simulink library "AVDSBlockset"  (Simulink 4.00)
undefined symbols (not defined in the file or in its folder): SimulinkConfiguration, SimulinkData, SimulinkVehicle01
libraries: simulink3 x7

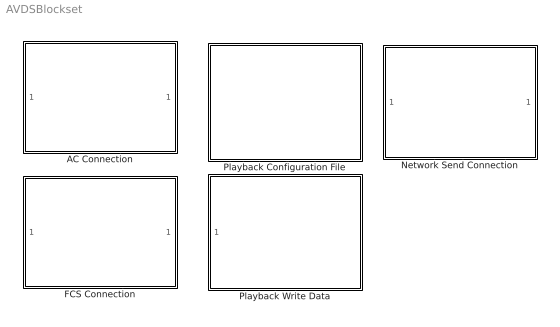
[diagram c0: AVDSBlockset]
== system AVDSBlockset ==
  AC Connection : Subsystem  Description=This block is used to connect Simulink to AVDS through the MATLAB AC model.  mask(AC Connection Block){RealTime=on}
      mask prompts: RealTime "Real Time Operation"
      mask help: This block connects a Simulink vehicle simulation to AVDS through shared memory. See help for more information.
  FCS Connection : Subsystem  Description=This block is used to connect Simulink to AVDS through the MATLAB AC model.
  Network Send Connection : Subsystem  Description=This block is used to connect Simulink to AVDS through the MATLAB AC model.  mask(Network Send Connection Block){VehicleHandleName=SimulinkVehicle01, TransmitRateHz=20, CraftType=1, InitLatitudeDeg=37.981523, InitLongitudeDeg=-122.063400, InitAltitudeFeet=10000, RealTime=on}
      mask prompts: VehicleHandleName "Vehicle Handle Name (up to 28 characters)"; TransmitRateHz "Transmit Rate (Hz)"; CraftType "Craft Type Index"; InitLatitudeDeg "Initial Latitude (Degrees Decimal)"; InitLongitudeDeg "Initial Longitude (Degrees Decimal) ( west longitude = negative)"; InitAltitudeFeet "Initial Altitude (Feet)"; RealTime "Real Time"
      mask help: Sends AVDS vehicle packets to the local network from Matlab using multicast network functions. See help for more information.
  Playback Configuration File : Subsystem  mask(Playback Configuration File Block){ConfigurationFileName=SimulinkConfiguration.ply.ini, DataFileNameBase=SimulinkData, NumberVehicles=10}
      mask prompts: ConfigurationFileName "Playback Configuration File Name"; DataFileNameBase "Data File Name Base (files use this name plus 2 digits)"; NumberVehicles "Number of Vehicles"
      mask help: This function writes an initialization file that configures AVDS playback. See help for more information.
  Playback Write Data : Subsystem  mask(Save Playback Data Block){DataFileNameBase=SimulinkData, VehicleID=01, NumberDataSignals=7}
      mask prompts: DataFileNameBase "Data File Name Base (files use this name plus the 2 digit ID)"; VehicleID "Vehicle ID (less than total number of vehicles)"; NumberDataSignals "Number Data Signals (number inputs to block)"
      mask help: Used to manage data for output to an AVDS playback file. See help for more information.

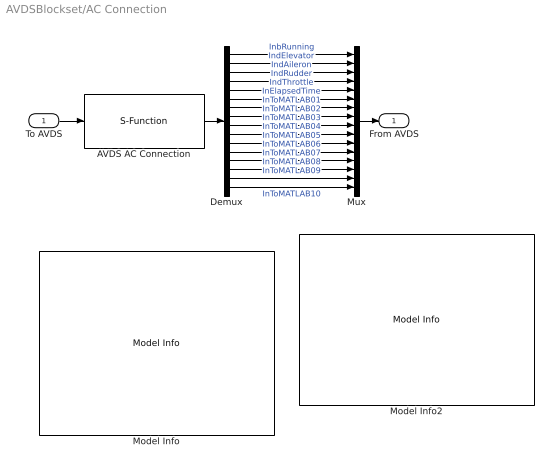
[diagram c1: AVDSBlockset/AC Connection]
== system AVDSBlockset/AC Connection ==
  To AVDS : Inport  Port=1  LatchInput=off
  AVDS AC Connection : S-Function  FunctionName=AVDSSimulationBlock  Parameters=3,25,4,16,RealTime  PortCounts=[]  SFunctionModules=''
  Demux : Demux  Outputs=16  BusSelectionMode=off
  Model Info : simulink3/Signals & Systems/Model Info  InitialBlockCM=none  BlockCM=none  Frame=off  DisplayStringWithTags=|  HorizontalTextAlignment=Left  LeftAlignmentValue=0.02  SourceBlockDiagram=AVDSBlockset  TagMaxNumber=20
      | Block Inputs:
      | OutPositionX, OutPositionY, OutPositionZ
      | OutRotationX, OutRotationY,OutRotationZ
      | OutAlpha, OutBeta
      | OutG
      | OutVelocity
      | OutM
      | OutDeltaRudde, OutDeltaElevator, OutDeltaAileron  
      | OutEngine
      | OutToAVDS01,  OutToAVDS02, OutToAVDS03
      | OutToAVDS04,  OutToAVDS05, OutToAVDS06,
      |  OutToAVDS07, OutToAVDS08,  OutToAVDS09,
      | OutToAVDS10
  Model Info2 : simulink3/Signals & Systems/Model Info  InitialBlockCM=none  BlockCM=none  Frame=off  DisplayStringWithTags=|  HorizontalTextAlignment=Left  LeftAlignmentValue=0.02  SourceBlockDiagram=AVDSBlockset  TagMaxNumber=20
      | BlockOutputs:
      | InbRunning
      | IndElevator, IndAileron, IndRudder, IndThrottle
      | InElapsedTime
      | InToMATLAB01, InToMATLAB02, InToMATLAB03
      | InToMATLAB04, InToMATLAB05, InToMATLAB06
      | InToMATLAB07, InToMATLAB08, InToMATLAB09
      | InToMATLAB10
  Mux : Mux  Inputs=16
  From AVDS : Outport  Port=1
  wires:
  To AVDS/1 -> AVDS AC Connection/1
  AVDS AC Connection/1 -> Demux/1
  Demux/1 -> Mux/1  "InbRunning"
  Demux/2 -> Mux/2  "IndElevator"
  Demux/3 -> Mux/3  "IndAileron"
  Demux/4 -> Mux/4  "IndRudder"
  Demux/5 -> Mux/5  "IndThrottle"
  Demux/6 -> Mux/6  "InElapsedTime"
  Demux/7 -> Mux/7  "InToMATLAB01"
  Demux/8 -> Mux/8  "InToMATLAB02"
  Demux/9 -> Mux/9  "InToMATLAB03"
  Demux/10 -> Mux/10  "InToMATLAB04"
  Demux/11 -> Mux/11  "InToMATLAB05"
  Demux/12 -> Mux/12  "InToMATLAB06"
  Demux/13 -> Mux/13  "InToMATLAB07"
  Demux/14 -> Mux/14  "InToMATLAB08"
  Demux/15 -> Mux/15  "InToMATLAB09"
  Demux/16 -> Mux/16  "InToMATLAB10"
  Mux/1 -> From AVDS/1

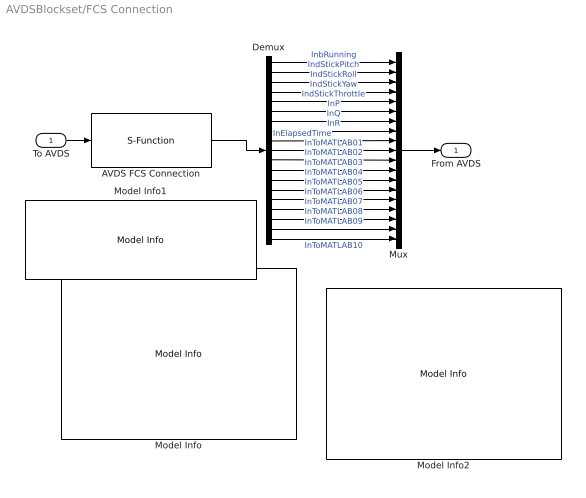
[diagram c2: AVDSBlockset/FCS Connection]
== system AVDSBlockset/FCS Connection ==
  To AVDS : Inport  Port=1  LatchInput=off
  AVDS FCS Connection : S-Function  FunctionName=AVDSSimulationBlock  Parameters=1,14,2,19  PortCounts=[]  SFunctionModules=''
  Demux : Demux  Outputs=19  BusSelectionMode=off
  Model Info : simulink3/Signals & Systems/Model Info  InitialBlockCM=none  BlockCM=none  Frame=off  DisplayStringWithTags=|  HorizontalTextAlignment=Left  LeftAlignmentValue=0.02  SourceBlockDiagram=AVDSBlockset  TagMaxNumber=20
      | Block Inputs:
      | 
      | OutPositionX, OutPositionY, OutPositionZ
      | OutRotationX, OutRotationY,OutRotationZ
      | OutAlpha, OutBeta
      | OutG
      | OutVelocity
      | OutM
      | OutDeltaRudde, OutDeltaElevator, OutDeltaAileron  
      | OutEngine
      | OutToAVDS01,  OutToAVDS02, OutToAVDS03
      | OutToAVDS04,  OutToAVDS05, OutToAVDS06,
      |  OutToAVDS07, OutToAVDS08,  OutToAVDS09,
      | OutToAVDS10
  Model Info1 : simulink3/Signals & Systems/Model Info  InitialBlockCM=none  BlockCM=none  Frame=off  DisplayStringWithTags=|  HorizontalTextAlignment=Left  LeftAlignmentValue=0.02  SourceBlockDiagram=AVDSBlockset  TagMaxNumber=20
      | AVDS AC Connection Block
      | 
      | Version %<ModelVersion>
      | Revision Date: %<LastModificationDate>
  Model Info2 : simulink3/Signals & Systems/Model Info  InitialBlockCM=none  BlockCM=none  Frame=off  DisplayStringWithTags=|  HorizontalTextAlignment=Left  LeftAlignmentValue=0.02  SourceBlockDiagram=AVDSBlockset  TagMaxNumber=20
      | BlockOutputs:
      | 
      | InbRunning
      | IndElevator, IndAileron, IndRudder, IndThrottle
      | InElapsedTime
      | InToMATLAB01, InToMATLAB02, InToMATLAB03
      | InToMATLAB04, InToMATLAB05, InToMATLAB06
      | InToMATLAB07, InToMATLAB08, InToMATLAB09
      | InToMATLAB10
  Mux : Mux  Inputs=19
  From AVDS : Outport  Port=1
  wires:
  AVDS FCS Connection/1 -> Demux/1
  To AVDS/1 -> AVDS FCS Connection/1
  Mux/1 -> From AVDS/1
  Demux/14 -> Mux/14  "InToMATLAB05"
  Demux/13 -> Mux/13  "InToMATLAB04"
  Demux/12 -> Mux/12  "InToMATLAB03"
  Demux/11 -> Mux/11  "InToMATLAB02"
  Demux/10 -> Mux/10  "InToMATLAB01"
  Demux/9 -> Mux/9  "InElapsedTime"
  Demux/8 -> Mux/8  "InR"
  Demux/7 -> Mux/7  "InQ"
  Demux/6 -> Mux/6  "InP"
  Demux/5 -> Mux/5  "IndStickThrottle"
  Demux/4 -> Mux/4  "IndStickYaw"
  Demux/3 -> Mux/3  "IndStickRoll"
  Demux/2 -> Mux/2  "IndStickPitch"
  Demux/1 -> Mux/1  "InbRunning"
  Demux/15 -> Mux/15  "InToMATLAB06"
  Demux/16 -> Mux/16  "InToMATLAB07"
  Demux/17 -> Mux/17  "InToMATLAB08"
  Demux/18 -> Mux/18  "InToMATLAB09"
  Demux/19 -> Mux/19  "InToMATLAB10"

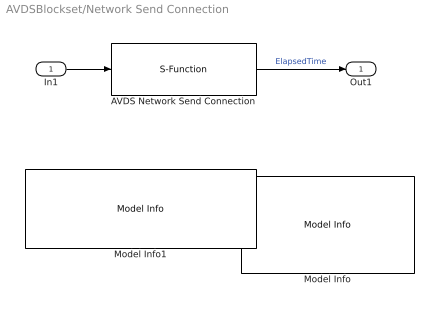
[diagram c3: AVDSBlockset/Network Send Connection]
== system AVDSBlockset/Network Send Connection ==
  In1 : Inport  Port=1  LatchInput=off
  AVDS Network Send Connection : S-Function  FunctionName=AVDSNetworkSendBlock  Parameters=VehicleHandleName,TransmitRateHz, CraftType, InitLatitudeDeg, InitLongitudeDeg, InitAltitudeFeet,RealTime  PortCounts=[]  SFunctionModules=''
  Model Info : simulink3/Signals & Systems/Model Info  InitialBlockCM=none  BlockCM=none  Frame=off  DisplayStringWithTags=|  HorizontalTextAlignment=Left  LeftAlignmentValue=0.02  SourceBlockDiagram=AVDSBlockset  TagMaxNumber=20
      | Block Inputs:
      | in_pos_X,in_pos_Y,in_pos_Z
      | ,in_rot_X,in_rot_Y,in_rot_Z
      | in_elev,in_ail,in_rud,in_engine
      | in_pos_dX,in_pos_dY,in_pos_dZ,
      | in_rot_dX,in_rot_dY,in_rot_dZ
  Model Info1 : simulink3/Signals & Systems/Model Info  InitialBlockCM=none  BlockCM=none  Frame=off  DisplayStringWithTags=|  HorizontalTextAlignment=Left  LeftAlignmentValue=0.02  SourceBlockDiagram=AVDSBlockset  TagMaxNumber=20
      | AVDS Network Connection Block
      | Version %<ModelVersion>
      | Revision Date: %<LastModificationDate>
  Out1 : Outport  Port=1
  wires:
  AVDS Network Send Connection/1 -> Out1/1  "ElapsedTime"
  In1/1 -> AVDS Network Send Connection/1

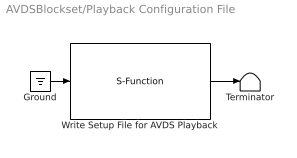
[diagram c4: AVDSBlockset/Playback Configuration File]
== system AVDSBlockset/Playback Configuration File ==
  Ground : Ground
  Terminator : Terminator
  Write Setup File for AVDS Playback : S-Function  FunctionName=AVDSPlaybackSetupBlock  Parameters=ConfigurationFileName,DataFileNameBase,NumberVehicles  PortCounts=[]  SFunctionModules=''
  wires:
  Write Setup File for AVDS Playback/1 -> Terminator/1
  Ground/1 -> Write Setup File for AVDS Playback/1

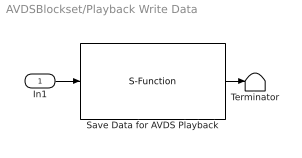
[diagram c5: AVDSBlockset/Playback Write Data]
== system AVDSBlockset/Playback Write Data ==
  In1 : Inport  Port=1  LatchInput=off
  Save Data for AVDS Playback : S-Function  FunctionName=AVDSPlaybackSaveBlock  Parameters=DataFileNameBase,VehicleID,NumberDataSignals  PortCounts=[]  SFunctionModules=''
  Terminator : Terminator
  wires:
  Save Data for AVDS Playback/1 -> Terminator/1
  In1/1 -> Save Data for AVDS Playback/1
